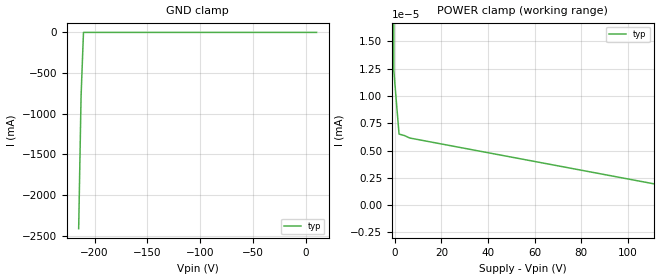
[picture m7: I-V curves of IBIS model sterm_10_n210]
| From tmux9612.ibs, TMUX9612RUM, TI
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| sterm_10_n210
[Model]   sterm_10_n210
Model_type   Terminator
|   typ   min   max
C_comp   2.533030e-12   NA   NA
[Voltage Range]   10_210   NA   NA
[Temperature Range]   27   NA   NA
[Power Clamp Reference]   10_210   NA   NA
[GND Clamp Reference]   0   NA   NA
[GND Clamp]
|   Voltage   I(typ)   I(min)   I(max)
-215V     -2.415A    NA         NA
-212.7V   -784.1mA   NA         NA
-210.5V   -102.8nA   NA         NA
10V       6.559nA    NA         NA
[POWER Clamp]
|   Voltage   I(typ)   I(min)   I(max)
-5V       1.055A     NA         NA
-2.727V   432.7mA    NA         NA
-454.5mV  12.37nA    NA         NA
1.818V    6.511nA    NA         NA
6.364V    6.153nA    NA         NA
220V      -2.413nA   NA         NA
